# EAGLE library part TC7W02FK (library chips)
NOR, 2-Array
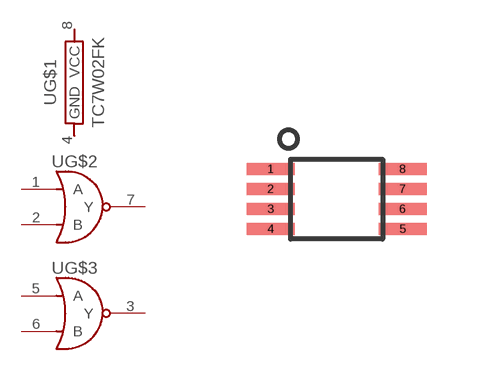
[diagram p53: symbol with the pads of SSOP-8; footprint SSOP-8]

Designator prefix U; gates G$1=SUPPLY G$2=NOR G$3=NOR

## TC7W02FK  [SSOP-8]
1  G$2:A
2  G$2:B
3  G$3:Y
4  G$1:GND
5  G$3:A
6  G$3:B
7  G$2:Y
8  G$1:VCC

## Footprint SSOP-8 (pad centres in mm)
smd 1.2 x 0.3: 1 -1.65,0.75; 2 -1.65,0.25; 3 -1.65,-0.25; 4 -1.65,-0.75; 5 1.65,-0.75; 6 1.65,-0.25; 7 1.65,0.25; 8 1.65,0.75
